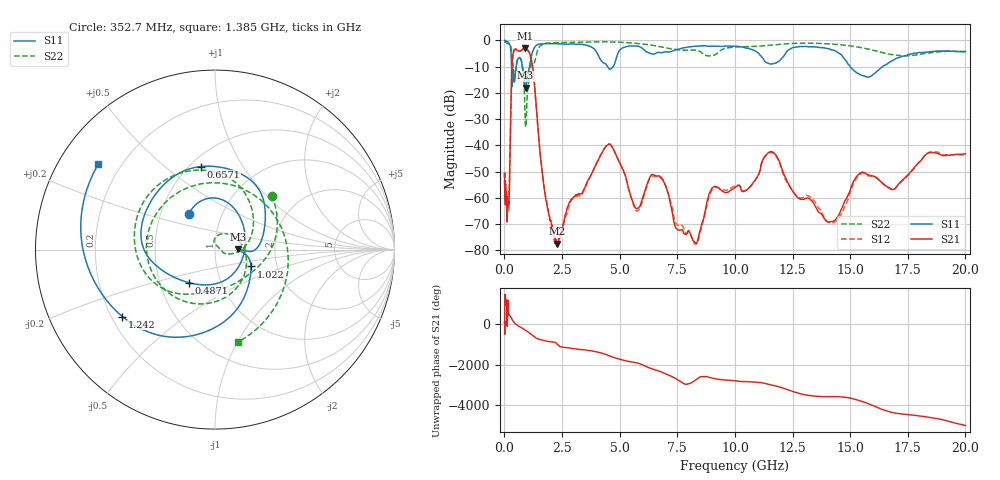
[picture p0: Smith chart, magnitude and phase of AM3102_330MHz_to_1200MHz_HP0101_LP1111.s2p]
! Date/Time: Tue, Sep 11, 2018 5:14 PM
! Network Analyzer: Agilent Technologies E8362B Rev: A.07.50.63
! Sweep from 0.010 to 20.000 GHz, 1601 Points, Sweep Type: LOG
! Power Supply: 4.949 V, 0.001 A
# Hz S DB R 50
!freq MagS11 AngS11 MagS21 AngS21 MagS12 AngS12 MagS22 AngS22
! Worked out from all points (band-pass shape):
!   1601 points, 10 MHz to 20 GHz, reference 50 ohm
!   highest |S21| = -3.03 dB at 890.6 MHz (marker M1); lowest = -77.4 dB at 2.303 GHz (marker M2)
!   |S21| within 3 dB of the highest: 362 MHz to 1.138 GHz (776.3 MHz wide, 103 % of centre)
!   lowest |S11| = -18.0 dB at 920.7 MHz (marker M3), VSWR 1.29, Z = 64.5 + j0.314 ohm
!   |S11| at or under -10 dB: 780.8 MHz to 1.088 GHz (307.2 MHz wide, 32.9 % of centre); 4.476 GHz to 4.712 GHz (235.4 MHz wide, 5.12 % of centre); 15.01 GHz to 16.4 GHz (1.398 GHz wide, 8.9 % of centre)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
!   |S22| runs from -32.9 to -0.3 dB; largest |S21 - S12| = 0.013
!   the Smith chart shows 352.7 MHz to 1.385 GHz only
!   S11 on the Smith chart (normalised r, x): 352.7 MHz: 0.69, +0.29; 487.1 MHz: 0.70, -0.28; 657.1 MHz: 0.57, +0.67; 1.022 GHz: 1.47, -0.29; 1.242 GHz: 0.24, -0.31; 1.385 GHz: 0.12, +0.32
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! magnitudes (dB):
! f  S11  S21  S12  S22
! 10 MHz  0.0  -50.7  -50.2  -0.3
! 35.55 MHz  0.0  -58.9  -57.8  -0.6
! 126.4 MHz  -0.4  -63.2  -63.2  -1.1
! 196.6 MHz  -1.1  -61.5  -63.6  -1.4
! 352.7 MHz  -12.2  -6.6  -6.7  -7.2
! 447.2 MHz  -15.1  -3.4  -3.5  -13.1
! 487.1 MHz  -12.6  -3.2  -3.3  -11.6
! 657.1 MHz  -6.6  -4.0  -4.2  -6.4
! 890.6 MHz  -17.0  -3.0  -3.1  -27.2
! 920.7 MHz  -18.0  -3.1  -3.2  -32.8
! 1.022 GHz  -13.1  -3.8  -3.8  -17.9
! 1.242 GHz  -3.9  -11.2  -11.3  -8.4
! 1.385 GHz  -1.9  -25.3  -25.7  -5.5
! 1.59 GHz  -1.4  -46.2  -46.1  -1.8
! 2.303 GHz  -1.3  -77.4  -77.4  -0.8
! 4.479 GHz  -10.0  -39.8  -39.6  -0.5
! 5.652 GHz  -2.1  -63.1  -63.9  -1.0
! 6.675 GHz  -4.5  -51.6  -51.9  -2.2
! 8.188 GHz  -2.2  -76.2  -76.6  -3.6
! 11.58 GHz  -8.9  -42.3  -42.7  -1.8
! 14.14 GHz  -3.4  -69.1  -69.6  -1.3
! 20 GHz  -4.3  -43.2  -43.8  -4.1
